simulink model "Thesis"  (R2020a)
settings: Solver=ode15s  StartTime=0.0  StopTime=1440  MaxStep=1  RelTol=1e-3
model workspace (MAT data in the model file):
  SDO_OutputTimes = [0 45 72 95 129 186 320 430 960 1290]
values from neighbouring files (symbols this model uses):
  BR = 5000    [VariablesHighBFloretsSR.m]    (also in VariablesHighBPowderSR.m; VariablesLowBFloretsSR.m; VariablesMedBFloretsSR.m; VariablesNoBFloretsSR.m)
  Cgl0 = 621.875    [VariablesHighBFloretsSR.m]    (also in VariablesHighBPowderSR.m = 383.33; VariablesLowBFloretsSR.m = 708.333; VariablesMedBFloretsSR.m = 667.70833; VariablesNoBFloretsSR.m = 734.375)
  ITC0 = 115.625    [VariablesHighBFloretsSR.m]    (also in VariablesHighBPowderSR.m = 354.17; VariablesLowBFloretsSR.m = 2.65154545455; VariablesMedBFloretsSR.m = 2.40689655172; VariablesNoBFloretsSR.m = 3.125)
  ka = 0.17952    [VariablesHighBFloretsSR.m]    (also in VariablesHighBPowderSR.m; VariablesLowBFloretsSR.m; VariablesMedBFloretsSR.m; VariablesNoBFloretsSR.m)
  ke = 0.024    [VariablesHighBFloretsSR.m]    (also in VariablesHighBPowderSR.m; VariablesLowBFloretsSR.m; VariablesMedBFloretsSR.m; VariablesNoBFloretsSR.m)
  keni = 0.0015    [VariablesHighBFloretsSR.m]    (also in VariablesHighBPowderSR.m; VariablesLowBFloretsSR.m; VariablesMedBFloretsSR.m; VariablesNoBFloretsSR.m)
  kf = 0.00333    [VariablesHighBFloretsSR.m]    (also in VariablesHighBPowderSR.m; VariablesLowBFloretsSR.m; VariablesMedBFloretsSR.m; VariablesNoBFloretsSR.m)
  Ki = 893.018606646    [VariablesHighBFloretsSR.m]    (also in VariablesHighBPowderSR.m; VariablesLowBFloretsSR.m; VariablesMedBFloretsSR.m; VariablesNoBFloretsSR.m)
  Km = 110.161136443    [VariablesHighBFloretsSR.m]    (also in VariablesHighBPowderSR.m; VariablesLowBFloretsSR.m; VariablesMedBFloretsSR.m; VariablesNoBFloretsSR.m)
  ktli = 0.002682    [VariablesHighBFloretsSR.m]    (also in VariablesHighBPowderSR.m; VariablesLowBFloretsSR.m; VariablesMedBFloretsSR.m; VariablesNoBFloretsSR.m)
  ktsi = 0.03518    [VariablesHighBFloretsSR.m]    (also in VariablesHighBPowderSR.m; VariablesLowBFloretsSR.m; VariablesMedBFloretsSR.m; VariablesNoBFloretsSR.m = 0.0351)
  M = 30    [VariablesHighBFloretsSR.m]    (also in VariablesHighBPowderSR.m; VariablesLowBFloretsSR.m; VariablesMedBFloretsSR.m; VariablesNoBFloretsSR.m)
  MYR = 0.0348960299    [VariablesHighBFloretsSR.m]    (also in VariablesHighBPowderSR.m; VariablesLowBFloretsSR.m = 0.000562839; VariablesMedBFloretsSR.m = 0.006528935; VariablesNoBFloretsSR.m = 1.12568e-05)
  NLI = 7    [VariablesHighBFloretsSR.m]    (also in VariablesHighBPowderSR.m; VariablesLowBFloretsSR.m; VariablesMedBFloretsSR.m; VariablesNoBFloretsSR.m)
  NSI = 6    [VariablesHighBFloretsSR.m]    (also in VariablesHighBPowderSR.m; VariablesLowBFloretsSR.m; VariablesMedBFloretsSR.m; VariablesNoBFloretsSR.m)
  SH = 0.02    [VariablesHighBFloretsSR.m]    (also in VariablesHighBPowderSR.m; VariablesLowBFloretsSR.m; VariablesMedBFloretsSR.m; VariablesNoBFloretsSR.m)
  SRR = 0.4737    [VariablesHighBFloretsSR.m]    (also in VariablesHighBPowderSR.m; VariablesLowBFloretsSR.m; VariablesMedBFloretsSR.m; VariablesNoBFloretsSR.m)
  St = 30    [VariablesHighBFloretsSR.m]    (also in VariablesHighBPowderSR.m; VariablesLowBFloretsSR.m; VariablesMedBFloretsSR.m; VariablesNoBFloretsSR.m)
  V1 = 0.096    [VariablesHighBFloretsSR.m]    (also in VariablesHighBPowderSR.m; VariablesLowBFloretsSR.m; VariablesMedBFloretsSR.m; VariablesNoBFloretsSR.m)
  V18 = 5    [VariablesHighBFloretsSR.m]    (also in VariablesHighBPowderSR.m; VariablesLowBFloretsSR.m; VariablesMedBFloretsSR.m; VariablesNoBFloretsSR.m)
  V2 = 0.05    [VariablesHighBFloretsSR.m]    (also in VariablesHighBPowderSR.m; VariablesLowBFloretsSR.m; VariablesMedBFloretsSR.m; VariablesNoBFloretsSR.m)
  V3 = 0.15    [VariablesHighBFloretsSR.m]    (also in VariablesHighBPowderSR.m; VariablesLowBFloretsSR.m; VariablesMedBFloretsSR.m; VariablesNoBFloretsSR.m)
  V4 = 0.2    [VariablesHighBFloretsSR.m]    (also in VariablesHighBPowderSR.m; VariablesLowBFloretsSR.m; VariablesMedBFloretsSR.m; VariablesNoBFloretsSR.m)
  VLI = 3.4    [VariablesHighBFloretsSR.m]    (also in VariablesHighBPowderSR.m; VariablesLowBFloretsSR.m; VariablesMedBFloretsSR.m; VariablesNoBFloretsSR.m)
  Vmax = 2070    [VariablesHighBFloretsSR.m]    (also in VariablesHighBPowderSR.m; VariablesLowBFloretsSR.m; VariablesMedBFloretsSR.m; VariablesNoBFloretsSR.m)
  VSI = 1.5    [VariablesHighBFloretsSR.m]    (also in VariablesHighBPowderSR.m; VariablesLowBFloretsSR.m; VariablesMedBFloretsSR.m; VariablesNoBFloretsSR.m)
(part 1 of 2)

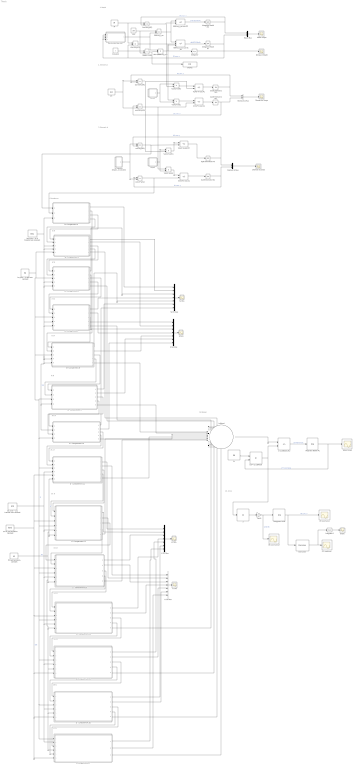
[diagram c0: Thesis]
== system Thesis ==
  note: 1. Mouth
  note: 2. Stomach a
  note: 3. Stomach b
  note: 4. Duodenum
  note: 5. SI
  note: 6. SI
  note: 7. SI
  note: 8. SI
  note: 9. SI
  note: 10. SI
  note: 11. LI
  note: 12. LI
  note: 13. LI
  note: 14. LI
  note: 15. LI
  note: 16. LI
  note: 17. LI
  note: 18. Blood
  note: 19. Urine
  -SRR*myr_rxn-out-nit,GL : Sum  Inputs=|---
  Blood Scope : Scope
  CL : Constant  Value=ke
  Constant : Constant
  Derivative : Derivative
  Display : Display
  Gain1 : Gain  Gain=V18
  ITC conc Urine : Scope
  ITC conc Urine2 : Scope
  ITC gut formation constant : Constant  Value=kf
  "ITC umol/min " : Scope
  In Blood : Sum  Inputs=|+++++++++++++
  Integrator : Integrator
  Integrator Blood ITC : Integrator
  Integrator Mouth GL : Integrator  InitialCondition=Cgl0
  Integrator Mouth ITC : Integrator  InitialCondition=ITC0
  Integrator Urine : Integrator
  Integrator1 : Integrator
  LI - Compartment 11 : Subsystem
  LI - Compartment 12 : Subsystem
  LI - Compartment 13 : Subsystem
  LI - Compartment 14 : Subsystem
  LI - Compartment 15 : Subsystem
  LI - Compartment 16 : Subsystem
  LI Compartment 17 : Subsystem
  LI GL Mux : Mux  Inputs=7
  LI GLs : Scope
  LI ITC Mux : Mux  Inputs=7
  LI ITCs : Scope
  M : Constant  Value=M
  Mouth Mux : Mux  Inputs=2
  Mouth Scope : Scope
  "Myrosinase Reaction " : Subsystem
  Nit=SRNR*myr_rxn : Product
  Nitriles in Mouth : Scope
  Out=M*y(GL) : Product
  Out=M*y(ITC) : Product
  "S, stomach emptying rate constant" : Subsystem
  SH : Constant  Value=SH
  SI - Compartment 10 : Subsystem
  SI - Compartment 5 : Subsystem
  SI - Compartment 6 : Subsystem
  SI - Compartment 7 : Subsystem
  SI - Compartment 8 : Subsystem
  SI - Compartment 9 : Subsystem
  SI GL Mux : Mux  Inputs=7
  SI GLs : Scope
  SI ITC Mux : Mux  Inputs=7
  SI ITCs : Scope
  "SI- Compartment 4 " : Subsystem
  SRNR=1-SRR : Sum  Inputs=+-
  SRR : Constant  Value=SRR
  SRR*myr_rxn : Product
  SRR*myr_rxn-out,ITC : Sum  Inputs=|+-
  Scope : Scope
  Stomach a Mux : Mux  Inputs=2
  Stomach a Scope : Scope
  Stomach b Mux : Mux  Inputs=2
  Stomach b Scope : Scope
  V1/V2 : Subsystem
  V1/V2*in(GL) : Product
  V1/V2*in(ITC) : Product
  V1/V2*in-out,GL : Sum  Inputs=|+-
  V1/V2*in-out,ITC : Sum  Inputs=+-
  V2/V3 : Subsystem
  V2/V3*in(GL) : Product
  V2/V3*in(ITC) : Product
  V2/V3*in-out,GL : Sum  Inputs=|+-
  V2/V3*in-out,ITC : Sum  Inputs=+-
  dy/dt Stomach1 GL1 : Integrator
  dy/dt Stomach1 ITC1 : Integrator
  dy/dt Stomach2 GL : Integrator
  dy/dt Stomach2 ITC : Integrator
  eru-ni gut formation constant : Constant  Value=keni
  in : Product  Inputs=1
  in-out(Blood,ITC) : Sum  Inputs=|+-
  ka,(min^-1) abs rate constant : Constant  Value=ka
  ktli,(min^-1) LI transfer rate constant : Constant  Value=ktli
  ktsi,(min^-1) SI transfer rate constant : Constant  Value=ktsi
  out= CL*y(Blood) : Product
  out=S*y(GL) : Product
  out=S*y(ITC) : Product
  out=SH*y(GL) : Product
  out=SH*y(ITC) : Product
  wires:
  Integrator Mouth ITC/1 -> Mouth Mux/1, Out=M*y(ITC)/2  "ITC conc, y"
  Integrator Mouth GL/1 -> Mouth Mux/2, Out=M*y(GL)/2, "Myrosinase Reaction "/1("GL conc, y"), "Myrosinase Reaction "/2("GL conc, y1"), "Myrosinase Reaction "/3("GL conc, y2")  "GL conc, y"
  Mouth Mux/1 -> Mouth Scope/1
  M/1 -> Out=M*y(GL)/1, Out=M*y(ITC)/1
  Out=M*y(ITC)/1 -> V1/V2*in(ITC)/2, SRR*myr_rxn-out,ITC/2
  "Myrosinase Reaction "/1(Out1) -> Nit=SRNR*myr_rxn/1, SRR*myr_rxn/2
  Out=M*y(GL)/1 -> -SRR*myr_rxn-out-nit,GL/2, V1/V2*in(GL)/1
  SRR*myr_rxn-out,ITC/1 -> Integrator Mouth ITC/1  "dy/dt ITC Mouth"
  -SRR*myr_rxn-out-nit,GL/1 -> Integrator Mouth GL/1  "dy/dt GL Mouth"
  SH/1 -> out=SH*y(ITC)/1, out=SH*y(GL)/2
  Stomach a Mux/1 -> Stomach a Scope/1
  dy/dt Stomach1 GL1/1 -> out=SH*y(GL)/1, Stomach a Mux/2  "GL conc, y"
  dy/dt Stomach1 ITC1/1 -> Stomach a Mux/1, out=SH*y(ITC)/2  "ITC conc, y"
  V1/V2/1(Out1) -> V1/V2*in(ITC)/1, V1/V2*in(GL)/2
  V1/V2*in(GL)/1 -> V1/V2*in-out,GL/1
  V1/V2*in(ITC)/1 -> V1/V2*in-out,ITC/1
  V1/V2*in-out,ITC/1 -> dy/dt Stomach1 ITC1/1
  V1/V2*in-out,GL/1 -> dy/dt Stomach1 GL1/1
  dy/dt Stomach2 GL/1 -> Stomach b Mux/2, out=S*y(GL)/1  "GL conc, y"
  V2/V3*in(ITC)/1 -> V2/V3*in-out,ITC/1
  out=SH*y(ITC)/1 -> V1/V2*in-out,ITC/2, V2/V3*in(ITC)/2
  dy/dt Stomach2 ITC/1 -> out=S*y(ITC)/2, Stomach b Mux/1  "ITC conc, y"
  out=SH*y(GL)/1 -> V2/V3*in(GL)/1, V1/V2*in-out,GL/2
  V2/V3*in(GL)/1 -> V2/V3*in-out,GL/1
  Stomach b Mux/1 -> Stomach b Scope/1
  V2/V3*in-out,GL/1 -> dy/dt Stomach2 GL/1
  V2/V3/1(Out1) -> V2/V3*in(ITC)/1, V2/V3*in(GL)/2
  V2/V3*in-out,ITC/1 -> dy/dt Stomach2 ITC/1
  "S, stomach emptying rate constant"/1(Out1) -> out=S*y(ITC)/1, out=S*y(GL)/2
  out=S*y(GL)/1 -> "SI- Compartment 4 "/2(In GL), V2/V3*in-out,GL/2
  out=S*y(ITC)/1 -> "SI- Compartment 4 "/1(In ITC), V2/V3*in-out,ITC/2
  SI ITC Mux/1 -> SI ITCs/1
  SI GL Mux/1 -> SI GLs/1
  "SI- Compartment 4 "/1("ITC conc, y") -> SI ITC Mux/1
  "SI- Compartment 4 "/2("GL conc, y") -> SI GL Mux/1
  "SI- Compartment 4 "/3(Out ITC) -> SI - Compartment 5/1(In ITC)
  "SI- Compartment 4 "/4(Out GL) -> SI - Compartment 5/2(In GL)
  SI - Compartment 5/1("ITC conc, y") -> SI ITC Mux/2
  SI - Compartment 5/2("GL conc, y") -> SI GL Mux/2
  SI - Compartment 5/3(Out ITC) -> SI - Compartment 6/1(In ITC)
  SI - Compartment 5/4(Out GL) -> SI - Compartment 6/2(In GL)
  SI - Compartment 6/1("ITC conc, y") -> SI ITC Mux/3
  SI - Compartment 6/2("GL conc, y") -> SI GL Mux/3
  SI - Compartment 6/3(Out ITC) -> SI - Compartment 7/1(In ITC)
  SI - Compartment 6/4(Out GL) -> SI - Compartment 7/2(In GL)
  SI - Compartment 7/1("ITC conc, y") -> SI ITC Mux/4
  SI - Compartment 7/2("GL conc, y") -> SI GL Mux/4
  ktsi,(min^-1) SI transfer rate constant/1 -> "SI- Compartment 4 "/3(ktsi), SI - Compartment 8/4(ktsi), SI - Compartment 10/2(ktsi), SI - Compartment 9/4(ktsi), SI - Compartment 8/5(ktsi1), SI - Compartment 7/5(ktsi GL), SI - Compartment 7/4(ktsi ITC), SI - Compartment 6/5(ktsi GL), SI - Compartment 6/4(ktsi ITC), SI - Compartment 5/4(ktsi GL), SI - Compartment 5/3(ktsi ITC)  "ktsi"
  SI - Compartment 7/3(Out ITC) -> SI - Compartment 8/1(In ITC)
  SI - Compartment 7/4(Out GL) -> SI - Compartment 8/2(In GL)
  SI - Compartment 8/1("ITC conc, y") -> SI ITC Mux/5
  SI - Compartment 8/2("GL conc, y") -> SI GL Mux/5
  SI - Compartment 8/3(Out ITC) -> SI - Compartment 9/1(In ITC)
  SI - Compartment 8/4(Out GL) -> SI - Compartment 9/2(In GL)
  SI - Compartment 9/1("ITC conc, y") -> SI ITC Mux/6
  SI - Compartment 9/2("GL conc, y") -> SI GL Mux/6
  LI GL Mux/1 -> LI GLs/1
  LI ITC Mux/1 -> LI ITCs/1
  SI - Compartment 9/3(Out ITC) -> SI - Compartment 10/1(In ITC)
  SI - Compartment 9/4(Out GL) -> SI - Compartment 10/3(In GL)
  SI - Compartment 10/1("ITC conc, y") -> SI ITC Mux/7
  SI - Compartment 10/2("GL conc, y") -> SI GL Mux/7
  SI - Compartment 10/3(Out ITC) -> LI - Compartment 11/1(In ITC)
  SI - Compartment 10/4(Out GL) -> LI - Compartment 11/2(In GL)
  LI - Compartment 11/1("ITC conc, y") -> LI ITC Mux/1
  LI - Compartment 11/2("GL conc, y") -> LI GL Mux/1
  LI - Compartment 11/3(Out ITC) -> LI - Compartment 12/1(In1)
  LI - Compartment 11/4(Out GL) -> LI - Compartment 12/2(In2)
  LI - Compartment 12/1("ITC conc, y") -> LI ITC Mux/2
  LI - Compartment 12/2("GL conc, y") -> LI GL Mux/2
  ktli,(min^-1) LI transfer rate constant/1 -> LI - Compartment 14/5(ktli), LI Compartment 17/2(ktli), LI - Compartment 16/4(ktli), LI - Compartment 15/4(ktli), LI - Compartment 13/5(ktli), LI - Compartment 12/5(ktli), LI - Compartment 11/4(ktli)  "ktli"
  ka,(min^-1) abs rate constant/1 -> SI - Compartment 7/3(ka), LI Compartment 17/1(ka), LI - Compartment 16/3(ka), LI - Compartment 15/3(ka), LI - Compartment 14/4(ka), LI - Compartment 13/4(ka), LI - Compartment 12/4(ka), LI - Compartment 11/3(ka), SI - Compartment 10/4(ka), SI - Compartment 9/3(ka), SI - Compartment 8/3(ka), SI - Compartment 6/3(ka), SI - Compartment 5/5(Ka)  "ka"
  eru-ni gut formation constant/1 -> LI Compartment 17/6(keni), LI - Compartment 16/6(keni), LI - Compartment 15/6(keni), LI - Compartment 14/3(keni), LI - Compartment 13/3(keni), LI - Compartment 11/5(keni), LI - Compartment 12/3(keni)  "keni"
  ITC gut formation constant/1 -> LI - Compartment 12/6(kf), LI - Compartment 11/6(kf), LI Compartment 17/4(kf), LI - Compartment 16/5(kf), LI - Compartment 15/5(kf), LI - Compartment 14/6(kf), LI - Compartment 13/6(kf)  "kf"
  LI - Compartment 12/3(Out ITC) -> LI - Compartment 13/1(In1)
  LI - Compartment 12/4(Out GL) -> LI - Compartment 13/2(In2)
  LI - Compartment 13/1("ITC conc, y") -> LI ITC Mux/3
  LI - Compartment 13/2("GL conc, y") -> LI GL Mux/3
  LI - Compartment 13/3(Out ITC) -> LI - Compartment 14/1(In1)
  LI - Compartment 13/4(Out GL) -> LI - Compartment 14/2(In2)
  LI - Compartment 14/1("ITC conc, y") -> LI ITC Mux/4
  LI - Compartment 14/2("GL conc, y") -> LI GL Mux/4
  LI - Compartment 14/3(Out ITC) -> LI - Compartment 15/1(In1)
  LI - Compartment 14/4(Out GL) -> LI - Compartment 15/2(In2)
  LI - Compartment 15/1("ITC conc, y") -> LI ITC Mux/5
  LI - Compartment 15/2("GL conc, y") -> LI GL Mux/5
  LI - Compartment 15/3(Out ITC) -> LI - Compartment 16/1(In1)
  LI - Compartment 15/4(Out GL) -> LI - Compartment 16/2(In2)
  LI - Compartment 16/1("ITC conc, y") -> LI ITC Mux/6
  LI - Compartment 16/2("GL conc, y") -> LI GL Mux/6
  LI - Compartment 16/3(Out ITC) -> LI Compartment 17/3(In3)
  LI - Compartment 16/4(Out GL) -> LI Compartment 17/5(In5)
  LI Compartment 17/1("ITC conc, y") -> LI ITC Mux/7
  LI Compartment 17/2("GL conc, y") -> LI GL Mux/7
  SI - Compartment 5/5(abs) -> In Blood/1
  SI - Compartment 6/5(abs) -> In Blood/2
  SI - Compartment 7/5(abs) -> In Blood/3
  SI - Compartment 8/5(abs) -> In Blood/4
  SI - Compartment 9/5(abs) -> In Blood/5
  SI - Compartment 10/5(abs) -> In Blood/6
  LI - Compartment 11/5(abs) -> In Blood/7
  LI - Compartment 12/5(abs) -> In Blood/8
  LI - Compartment 13/5(abs) -> In Blood/9
  LI - Compartment 14/5(abs) -> In Blood/10
  LI - Compartment 15/5(abs) -> In Blood/11
  LI Compartment 17/3(abs) -> In Blood/13
  In Blood/1 -> in-out(Blood,ITC)/1
  CL/1 -> out= CL*y(Blood)/1
  Integrator Blood ITC/1 -> Blood Scope/1, out= CL*y(Blood)/2  "ITC conc Blood"
  out= CL*y(Blood)/1 -> in-out(Blood,ITC)/2, in/1
  in-out(Blood,ITC)/1 -> Integrator Blood ITC/1  "dy/dt Blood ITC"
  in/1 -> Gain1/1
  Integrator Urine/1 -> Derivative/1, ITC conc Urine/1  "ITC conc, y"
  LI - Compartment 16/5(abs) -> In Blood/12
  Gain1/1 -> ITC conc Urine2/1, Integrator Urine/1  "umol ITC"
  Derivative/1 -> Integrator1/1, "ITC umol/min "/1
  Nit=SRNR*myr_rxn/1 -> -SRR*myr_rxn-out-nit,GL/3, Integrator/1
  Integrator/1 -> Nitriles in Mouth/1
  Integrator1/1 -> Scope/1
  SRR/1 -> SRR*myr_rxn/1, SRNR=1-SRR/2
  SRR*myr_rxn/1 -> SRR*myr_rxn-out,ITC/1, -SRR*myr_rxn-out-nit,GL/1
  Constant/1 -> SRNR=1-SRR/1
  SRNR=1-SRR/1 -> Display/1, Nit=SRNR*myr_rxn/2

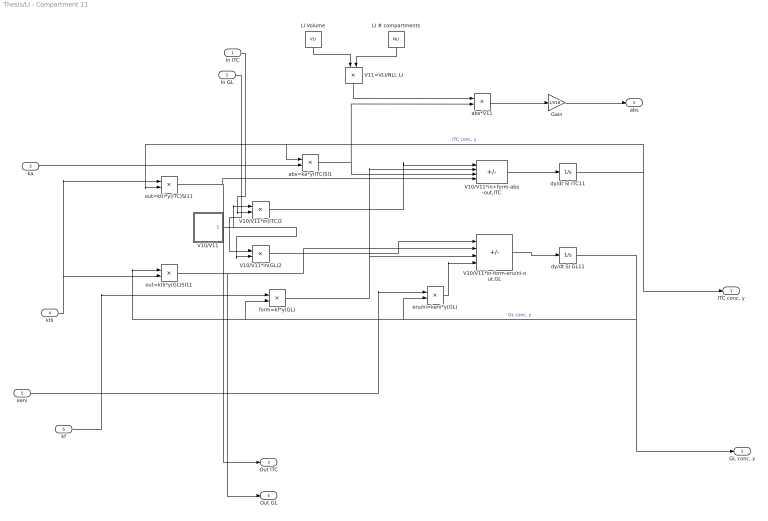
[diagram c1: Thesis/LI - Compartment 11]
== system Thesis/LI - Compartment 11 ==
  In ITC : Inport
  In GL : Inport  Port=2
  ka : Inport  Port=3
  ktli : Inport  Port=4
  keni : Inport  Port=5
  kf : Inport  Port=6
  Gain : Gain  Gain=1/V18
  LI # compartments : Constant  Value=NLI
  LI Volume : Constant  Value=VLI
  V10/V11 : Subsystem
  V10/V11*in(GL)2 : Product
  V10/V11*in(ITC)2 : Product
  V10/V11*in+form-abs-out,ITC : Sum  Inputs=++--
  V10/V11*in-form-eru/ni-out,GL : Sum  Inputs=|+---
  "V11=VLI/NLI, LI " : Product  Inputs=*/
  abs*V11 : Product
  abs=ka*y(ITC)SI1 : Product
  dy/dt SI GL11 : Integrator
  dy/dt SI ITC11 : Integrator
  eru/ni=keni*y(GL) : Product
  form=kf*y(GL) : Product
  out=ktli*y(GL)SI11 : Product
  out=ktli*y(ITC)SI11 : Product
  "ITC conc, y" : Outport
  "GL conc, y" : Outport  Port=2
  Out ITC : Outport  Port=3
  Out GL : Outport  Port=4
  abs : Outport  Port=5
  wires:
  dy/dt SI ITC11/1 -> "ITC conc, y"/1, abs=ka*y(ITC)SI1/1, out=ktli*y(ITC)SI11/2  "ITC conc, y"
  abs=ka*y(ITC)SI1/1 -> abs*V11/2, V10/V11*in+form-abs-out,ITC/3
  out=ktli*y(GL)SI11/1 -> Out GL/1, V10/V11*in-form-eru/ni-out,GL/2
  V10/V11*in-form-eru/ni-out,GL/1 -> dy/dt SI GL11/1
  dy/dt SI GL11/1 -> form=kf*y(GL)/2, out=ktli*y(GL)SI11/1, eru/ni=keni*y(GL)/2, "GL conc, y"/1  "GL conc, y"
  ktli/1 -> out=ktli*y(GL)SI11/2, out=ktli*y(ITC)SI11/1
  V10/V11*in(GL)2/1 -> V10/V11*in-form-eru/ni-out,GL/1
  V10/V11/1(Out1) -> V10/V11*in(GL)2/2, V10/V11*in(ITC)2/1
  form=kf*y(GL)/1 -> V10/V11*in+form-abs-out,ITC/2, V10/V11*in-form-eru/ni-out,GL/3
  V10/V11*in(ITC)2/1 -> V10/V11*in+form-abs-out,ITC/1
  V10/V11*in+form-abs-out,ITC/1 -> dy/dt SI ITC11/1
  eru/ni=keni*y(GL)/1 -> V10/V11*in-form-eru/ni-out,GL/4
  out=ktli*y(ITC)SI11/1 -> Out ITC/1, V10/V11*in+form-abs-out,ITC/4
  ka/1 -> abs=ka*y(ITC)SI1/2
  In ITC/1 -> V10/V11*in(ITC)2/2
  In GL/1 -> V10/V11*in(GL)2/1
  keni/1 -> eru/ni=keni*y(GL)/1
  kf/1 -> form=kf*y(GL)/1
  LI Volume/1 -> "V11=VLI/NLI, LI "/1
  LI # compartments/1 -> "V11=VLI/NLI, LI "/2
  "V11=VLI/NLI, LI "/1 -> abs*V11/1
  abs*V11/1 -> Gain/1
  Gain/1 -> abs/1

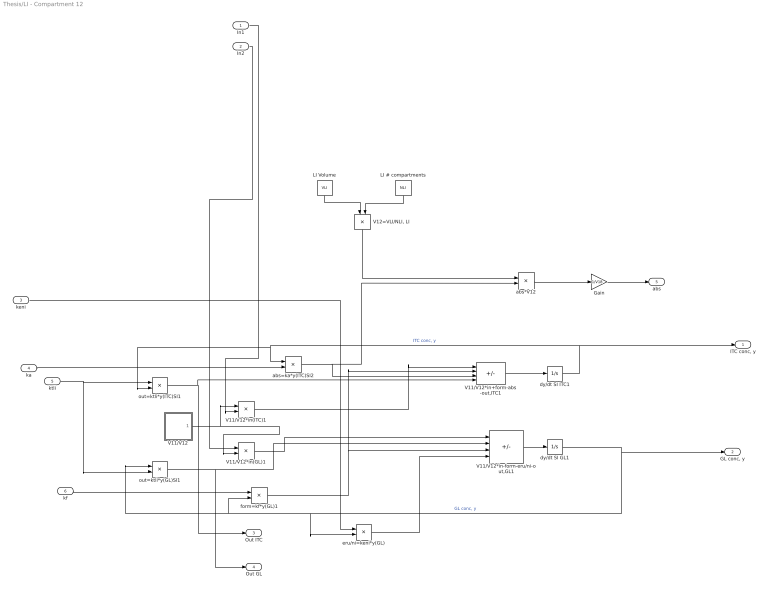
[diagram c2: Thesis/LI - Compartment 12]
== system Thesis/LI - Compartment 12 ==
  In1 : Inport
  In2 : Inport  Port=2
  keni : Inport  Port=3
  ka : Inport  Port=4
  ktli : Inport  Port=5
  kf : Inport  Port=6
  Gain : Gain  Gain=1/V18
  LI # compartments : Constant  Value=NLI
  LI Volume : Constant  Value=VLI
  V11/V12 : Subsystem
  V11/V12*in(GL)1 : Product
  V11/V12*in(ITC)1 : Product
  V11/V12*in+form-abs-out,ITC1 : Sum  Inputs=++--
  V11/V12*in-form-eru/ni-out,GL1 : Sum  Inputs=|+---
  "V12=VLI/NLI, LI " : Product  Inputs=*/
  abs*V12 : Product
  abs=ka*y(ITC)SI2 : Product
  dy/dt SI GL1 : Integrator
  dy/dt SI ITC1 : Integrator
  eru/ni=keni*y(GL) : Product
  form=kf*y(GL)1 : Product
  out=ktli*y(GL)SI1 : Product
  out=ktli*y(ITC)SI1 : Product
  "ITC conc, y" : Outport
  "GL conc, y" : Outport  Port=2
  Out ITC : Outport  Port=3
  Out GL : Outport  Port=4
  abs : Outport  Port=5
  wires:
  In2/1 -> V11/V12*in(GL)1/1
  dy/dt SI GL1/1 -> "GL conc, y"/1, form=kf*y(GL)1/2, out=ktli*y(GL)SI1/1, eru/ni=keni*y(GL)/2  "GL conc, y"
  V11/V12/1(Out1) -> V11/V12*in(GL)1/2, V11/V12*in(ITC)1/1
  dy/dt SI ITC1/1 -> "ITC conc, y"/1, abs=ka*y(ITC)SI2/1, out=ktli*y(ITC)SI1/2  "ITC conc, y"
  eru/ni=keni*y(GL)/1 -> V11/V12*in-form-eru/ni-out,GL1/4
  V11/V12*in-form-eru/ni-out,GL1/1 -> dy/dt SI GL1/1
  keni/1 -> eru/ni=keni*y(GL)/1
  V11/V12*in(GL)1/1 -> V11/V12*in-form-eru/ni-out,GL1/1
  ktli/1 -> out=ktli*y(GL)SI1/2, out=ktli*y(ITC)SI1/1
  out=ktli*y(GL)SI1/1 -> Out GL/1, V11/V12*in-form-eru/ni-out,GL1/2
  form=kf*y(GL)1/1 -> V11/V12*in+form-abs-out,ITC1/2, V11/V12*in-form-eru/ni-out,GL1/3
  out=ktli*y(ITC)SI1/1 -> Out ITC/1, V11/V12*in+form-abs-out,ITC1/4
  V11/V12*in+form-abs-out,ITC1/1 -> dy/dt SI ITC1/1
  V11/V12*in(ITC)1/1 -> V11/V12*in+form-abs-out,ITC1/1
  ka/1 -> abs=ka*y(ITC)SI2/2
  In1/1 -> V11/V12*in(ITC)1/2
  kf/1 -> form=kf*y(GL)1/1
  LI # compartments/1 -> "V12=VLI/NLI, LI "/2
  LI Volume/1 -> "V12=VLI/NLI, LI "/1
  abs*V12/1 -> Gain/1
  Gain/1 -> abs/1
  abs=ka*y(ITC)SI2/1 -> abs*V12/2, V11/V12*in+form-abs-out,ITC1/3
  "V12=VLI/NLI, LI "/1 -> abs*V12/1

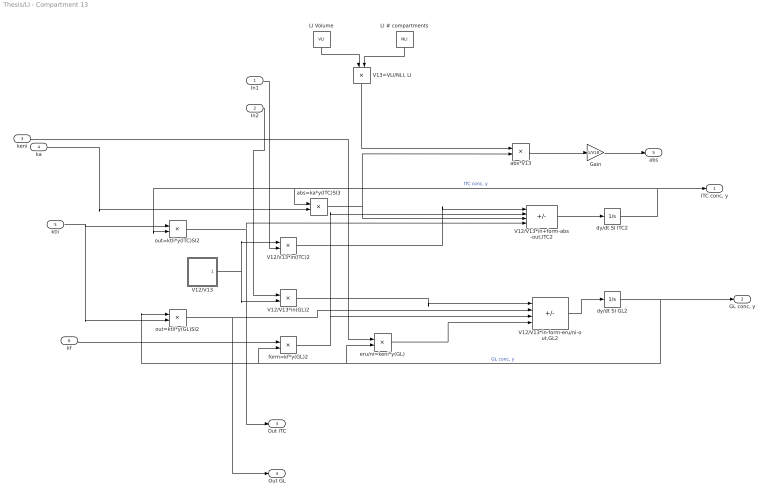
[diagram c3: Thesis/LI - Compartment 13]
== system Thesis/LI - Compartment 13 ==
  In1 : Inport
  In2 : Inport  Port=2
  keni : Inport  Port=3
  ka : Inport  Port=4
  ktli : Inport  Port=5
  kf : Inport  Port=6
  Gain : Gain  Gain=1/V18
  LI # compartments : Constant  Value=NLI
  LI Volume : Constant  Value=VLI
  V12/V13 : Subsystem
  V12/V13*in(GL)2 : Product
  V12/V13*in(ITC)2 : Product
  V12/V13*in+form-abs-out,ITC2 : Sum  Inputs=++--
  V12/V13*in-form-eru/ni-out,GL2 : Sum  Inputs=|+---
  "V13=VLI/NLI, LI " : Product  Inputs=*/
  abs*V13 : Product
  abs=ka*y(ITC)SI3 : Product
  dy/dt SI GL2 : Integrator
  dy/dt SI ITC2 : Integrator
  eru/ni=keni*y(GL) : Product
  form=kf*y(GL)2 : Product
  out=ktli*y(GL)SI2 : Product
  out=ktli*y(ITC)SI2 : Product
  "ITC conc, y" : Outport
  "GL conc, y" : Outport  Port=2
  Out ITC : Outport  Port=3
  Out GL : Outport  Port=4
  abs : Outport  Port=5
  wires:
  dy/dt SI GL2/1 -> "GL conc, y"/1, form=kf*y(GL)2/2, out=ktli*y(GL)SI2/1, eru/ni=keni*y(GL)/2  "GL conc, y"
  eru/ni=keni*y(GL)/1 -> V12/V13*in-form-eru/ni-out,GL2/4
  out=ktli*y(GL)SI2/1 -> Out GL/1, V12/V13*in-form-eru/ni-out,GL2/2
  V12/V13*in(GL)2/1 -> V12/V13*in-form-eru/ni-out,GL2/1
  out=ktli*y(ITC)SI2/1 -> Out ITC/1, V12/V13*in+form-abs-out,ITC2/4
  V12/V13/1(Out1) -> V12/V13*in(GL)2/2, V12/V13*in(ITC)2/1
  keni/1 -> eru/ni=keni*y(GL)/1
  V12/V13*in-form-eru/ni-out,GL2/1 -> dy/dt SI GL2/1
  dy/dt SI ITC2/1 -> abs=ka*y(ITC)SI3/1, out=ktli*y(ITC)SI2/2, "ITC conc, y"/1  "ITC conc, y"
  ka/1 -> abs=ka*y(ITC)SI3/2
  V12/V13*in+form-abs-out,ITC2/1 -> dy/dt SI ITC2/1
  V12/V13*in(ITC)2/1 -> V12/V13*in+form-abs-out,ITC2/1
  form=kf*y(GL)2/1 -> V12/V13*in+form-abs-out,ITC2/2, V12/V13*in-form-eru/ni-out,GL2/3
  In2/1 -> V12/V13*in(GL)2/1
  ktli/1 -> out=ktli*y(GL)SI2/2, out=ktli*y(ITC)SI2/1
  In1/1 -> V12/V13*in(ITC)2/2
  kf/1 -> form=kf*y(GL)2/1
  LI # compartments/1 -> "V13=VLI/NLI, LI "/2
  LI Volume/1 -> "V13=VLI/NLI, LI "/1
  abs*V13/1 -> Gain/1
  Gain/1 -> abs/1
  abs=ka*y(ITC)SI3/1 -> abs*V13/2, V12/V13*in+form-abs-out,ITC2/3
  "V13=VLI/NLI, LI "/1 -> abs*V13/1

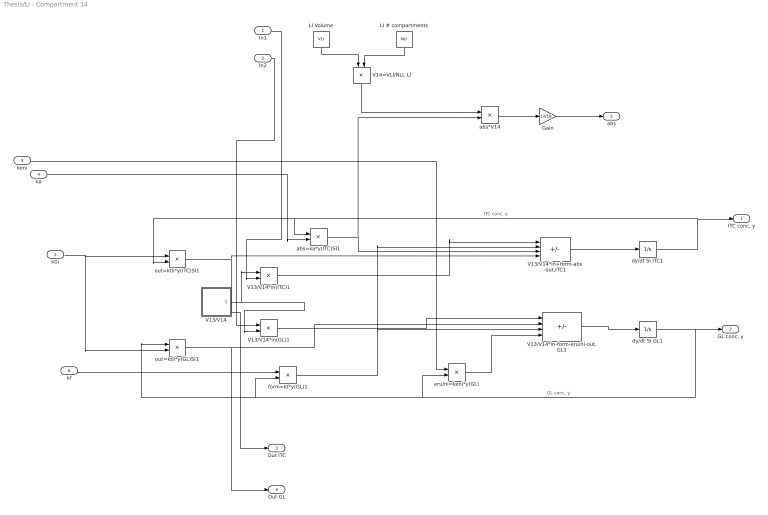
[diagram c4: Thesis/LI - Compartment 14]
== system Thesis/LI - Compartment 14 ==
  In1 : Inport
  In2 : Inport  Port=2
  keni : Inport  Port=3
  ka : Inport  Port=4
  ktli : Inport  Port=5
  kf : Inport  Port=6
  Gain : Gain  Gain=1/V18
  LI # compartments : Constant  Value=NLI
  LI Volume : Constant  Value=VLI
  V13/V14 : Subsystem
  V13/V14*in(GL)1 : Product
  V13/V14*in(ITC)1 : Product
  V13/V14*in+form-abs-out,ITC1 : Sum  Inputs=++--
  V13/V14*in-form-eru/ni-out,GL1 : Sum  Inputs=|+---
  "V14=VLI/NLI, LI " : Product  Inputs=*/
  abs*V14 : Product
  abs=ka*y(ITC)SI1 : Product
  dy/dt SI GL1 : Integrator
  dy/dt SI ITC1 : Integrator
  eru/ni=keni*y(GL) : Product
  form=kf*y(GL)1 : Product
  out=ktli*y(GL)SI1 : Product
  out=ktli*y(ITC)SI1 : Product
  "ITC conc, y" : Outport
  "GL conc, y" : Outport  Port=2
  Out ITC : Outport  Port=3
  Out GL : Outport  Port=4
  abs : Outport  Port=5
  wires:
  V13/V14/1(Out1) -> V13/V14*in(GL)1/2, V13/V14*in(ITC)1/1
  out=ktli*y(GL)SI1/1 -> Out GL/1, V13/V14*in-form-eru/ni-out,GL1/2
  dy/dt SI ITC1/1 -> abs=ka*y(ITC)SI1/1, out=ktli*y(ITC)SI1/2, "ITC conc, y"/1  "ITC conc, y"
  V13/V14*in(ITC)1/1 -> V13/V14*in+form-abs-out,ITC1/1
  out=ktli*y(ITC)SI1/1 -> V13/V14*in+form-abs-out,ITC1/4, Out ITC/1
  form=kf*y(GL)1/1 -> V13/V14*in+form-abs-out,ITC1/2, V13/V14*in-form-eru/ni-out,GL1/3
  eru/ni=keni*y(GL)/1 -> V13/V14*in-form-eru/ni-out,GL1/4
  V13/V14*in+form-abs-out,ITC1/1 -> dy/dt SI ITC1/1
  V13/V14*in(GL)1/1 -> V13/V14*in-form-eru/ni-out,GL1/1
  V13/V14*in-form-eru/ni-out,GL1/1 -> dy/dt SI GL1/1
  dy/dt SI GL1/1 -> "GL conc, y"/1, form=kf*y(GL)1/2, out=ktli*y(GL)SI1/1, eru/ni=keni*y(GL)/2  "GL conc, y"
  In2/1 -> V13/V14*in(GL)1/1
  ka/1 -> abs=ka*y(ITC)SI1/2
  keni/1 -> eru/ni=keni*y(GL)/1
  In1/1 -> V13/V14*in(ITC)1/2
  kf/1 -> form=kf*y(GL)1/1
  ktli/1 -> out=ktli*y(GL)SI1/2, out=ktli*y(ITC)SI1/1
  LI # compartments/1 -> "V14=VLI/NLI, LI "/2
  LI Volume/1 -> "V14=VLI/NLI, LI "/1
  abs*V14/1 -> Gain/1
  Gain/1 -> abs/1
  abs=ka*y(ITC)SI1/1 -> abs*V14/2, V13/V14*in+form-abs-out,ITC1/3
  "V14=VLI/NLI, LI "/1 -> abs*V14/1

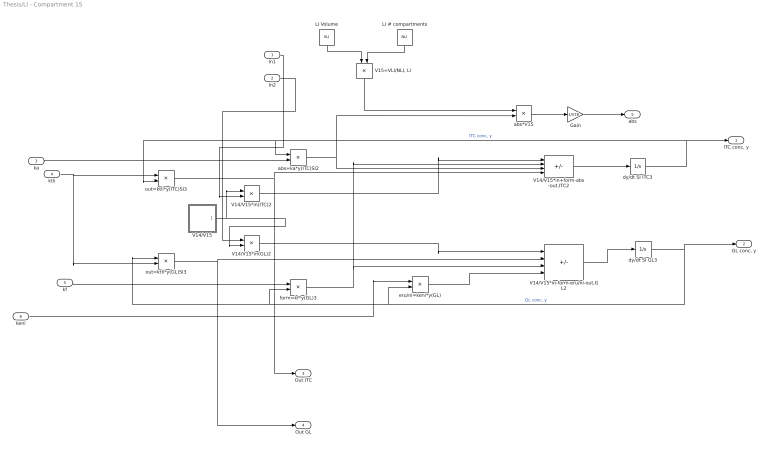
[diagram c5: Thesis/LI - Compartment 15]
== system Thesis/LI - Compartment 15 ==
  In1 : Inport
  In2 : Inport  Port=2
  ka : Inport  Port=3
  ktli : Inport  Port=4
  kf : Inport  Port=5
  keni : Inport  Port=6
  Gain : Gain  Gain=1/V18
  LI # compartments : Constant  Value=NLI
  LI Volume : Constant  Value=VLI
  V14/V15 : Subsystem
  V14/V15*in(GL)2 : Product
  V14/V15*in(ITC)2 : Product
  V14/V15*in+form-abs-out,ITC2 : Sum  Inputs=++--
  V14/V15*in-form-eru/ni-out,GL2 : Sum  Inputs=|+---
  "V15=VLI/NLI, LI " : Product  Inputs=*/
  abs*V15 : Product
  abs=ka*y(ITC)SI2 : Product
  dy/dt SI GL3 : Integrator
  dy/dt SI ITC3 : Integrator
  eru/ni=keni*y(GL) : Product
  form=kf*y(GL)3 : Product
  out=ktli*y(GL)SI3 : Product
  out=ktli*y(ITC)SI3 : Product
  "ITC conc, y" : Outport
  "GL conc, y" : Outport  Port=2
  Out ITC : Outport  Port=3
  Out GL : Outport  Port=4
  abs : Outport  Port=5
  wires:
  In2/1 -> V14/V15*in(GL)2/1
  V14/V15*in(GL)2/1 -> V14/V15*in-form-eru/ni-out,GL2/1
  dy/dt SI GL3/1 -> "GL conc, y"/1, form=kf*y(GL)3/2, out=ktli*y(GL)SI3/1, eru/ni=keni*y(GL)/2  "GL conc, y"
  eru/ni=keni*y(GL)/1 -> V14/V15*in-form-eru/ni-out,GL2/4
  out=ktli*y(GL)SI3/1 -> Out GL/1, V14/V15*in-form-eru/ni-out,GL2/2
  out=ktli*y(ITC)SI3/1 -> Out ITC/1, V14/V15*in+form-abs-out,ITC2/4
  dy/dt SI ITC3/1 -> abs=ka*y(ITC)SI2/1, out=ktli*y(ITC)SI3/2, "ITC conc, y"/1  "ITC conc, y"
  V14/V15/1(Out1) -> V14/V15*in(GL)2/2, V14/V15*in(ITC)2/1
  keni/1 -> eru/ni=keni*y(GL)/1
  V14/V15*in-form-eru/ni-out,GL2/1 -> dy/dt SI GL3/1
  ka/1 -> abs=ka*y(ITC)SI2/2
  V14/V15*in+form-abs-out,ITC2/1 -> dy/dt SI ITC3/1
  form=kf*y(GL)3/1 -> V14/V15*in+form-abs-out,ITC2/2, V14/V15*in-form-eru/ni-out,GL2/3
  kf/1 -> form=kf*y(GL)3/1
  V14/V15*in(ITC)2/1 -> V14/V15*in+form-abs-out,ITC2/1
  ktli/1 -> out=ktli*y(GL)SI3/2, out=ktli*y(ITC)SI3/1
  In1/1 -> V14/V15*in(ITC)2/2
  LI # compartments/1 -> "V15=VLI/NLI, LI "/2
  LI Volume/1 -> "V15=VLI/NLI, LI "/1
  abs*V15/1 -> Gain/1
  Gain/1 -> abs/1
  abs=ka*y(ITC)SI2/1 -> V14/V15*in+form-abs-out,ITC2/3, abs*V15/2
  "V15=VLI/NLI, LI "/1 -> abs*V15/1

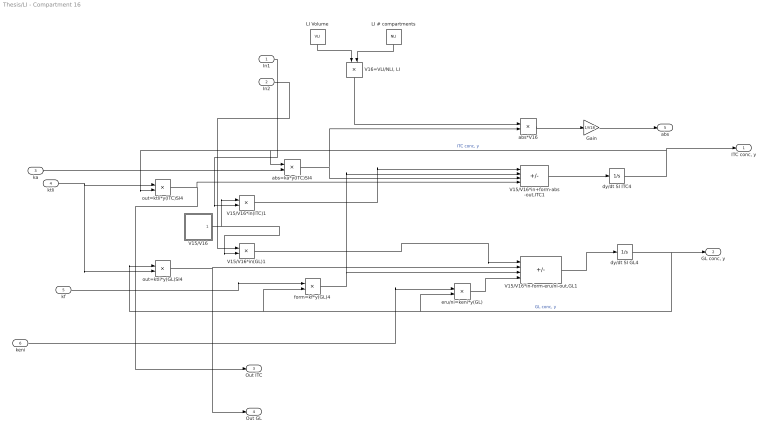
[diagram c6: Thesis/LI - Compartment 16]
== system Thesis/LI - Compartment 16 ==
  In1 : Inport
  In2 : Inport  Port=2
  ka : Inport  Port=3
  ktli : Inport  Port=4
  kf : Inport  Port=5
  keni : Inport  Port=6
  Gain : Gain  Gain=1/V18
  LI # compartments : Constant  Value=NLI
  LI Volume : Constant  Value=VLI
  V15/V16 : Subsystem
  V15/V16*in(GL)1 : Product
  V15/V16*in(ITC)1 : Product
  V15/V16*in+form-abs-out,ITC1 : Sum  Inputs=++--
  V15/V16*in-form-eru/ni-out,GL1 : Sum  Inputs=|+---
  "V16=VLI/NLI, LI " : Product  Inputs=*/
  abs*V16 : Product
  abs=ka*y(ITC)SI4 : Product
  dy/dt SI GL4 : Integrator
  dy/dt SI ITC4 : Integrator
  eru/ni=keni*y(GL) : Product
  form=kf*y(GL)4 : Product
  out=ktli*y(GL)SI4 : Product
  out=ktli*y(ITC)SI4 : Product
  "ITC conc, y" : Outport
  "GL conc, y" : Outport  Port=2
  Out ITC : Outport  Port=3
  Out GL : Outport  Port=4
  abs : Outport  Port=5
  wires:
  out=ktli*y(ITC)SI4/1 -> Out ITC/1, V15/V16*in+form-abs-out,ITC1/4
  out=ktli*y(GL)SI4/1 -> Out GL/1, V15/V16*in-form-eru/ni-out,GL1/2
  dy/dt SI ITC4/1 -> abs=ka*y(ITC)SI4/1, out=ktli*y(ITC)SI4/2, "ITC conc, y"/1  "ITC conc, y"
  V15/V16*in(ITC)1/1 -> V15/V16*in+form-abs-out,ITC1/1
  ka/1 -> abs=ka*y(ITC)SI4/2
  dy/dt SI GL4/1 -> "GL conc, y"/1, form=kf*y(GL)4/2, out=ktli*y(GL)SI4/1, eru/ni=keni*y(GL)/2  "GL conc, y"
  In1/1 -> V15/V16*in(ITC)1/2
  V15/V16/1(Out1) -> V15/V16*in(GL)1/2, V15/V16*in(ITC)1/1
  V15/V16*in+form-abs-out,ITC1/1 -> dy/dt SI ITC4/1
  V15/V16*in-form-eru/ni-out,GL1/1 -> dy/dt SI GL4/1
  keni/1 -> eru/ni=keni*y(GL)/1
  eru/ni=keni*y(GL)/1 -> V15/V16*in-form-eru/ni-out,GL1/4
  V15/V16*in(GL)1/1 -> V15/V16*in-form-eru/ni-out,GL1/1
  form=kf*y(GL)4/1 -> V15/V16*in+form-abs-out,ITC1/2, V15/V16*in-form-eru/ni-out,GL1/3
  In2/1 -> V15/V16*in(GL)1/1
  kf/1 -> form=kf*y(GL)4/1
  ktli/1 -> out=ktli*y(GL)SI4/2, out=ktli*y(ITC)SI4/1
  LI # compartments/1 -> "V16=VLI/NLI, LI "/2
  LI Volume/1 -> "V16=VLI/NLI, LI "/1
  abs*V16/1 -> Gain/1
  Gain/1 -> abs/1
  abs=ka*y(ITC)SI4/1 -> abs*V16/2, V15/V16*in+form-abs-out,ITC1/3
  "V16=VLI/NLI, LI "/1 -> abs*V16/1

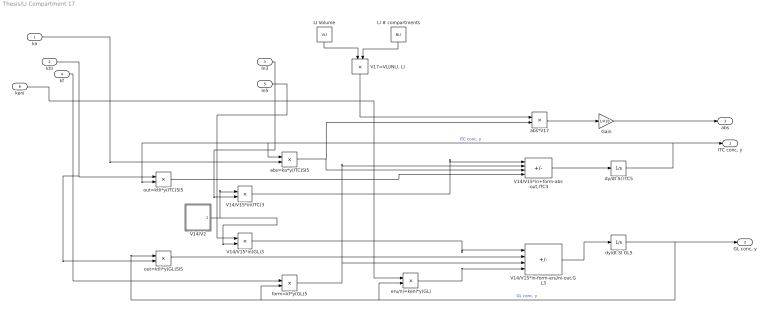
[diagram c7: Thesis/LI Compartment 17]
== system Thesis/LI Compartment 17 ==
  ka : Inport
  ktli : Inport  Port=2
  In3 : Inport  Port=3
  kf : Inport  Port=4
  In5 : Inport  Port=5
  keni : Inport  Port=6
  Gain : Gain  Gain=1/V18
  LI # compartments : Constant  Value=NLI
  LI Volume : Constant  Value=VLI
  V14/V15*in(GL)3 : Product
  V14/V15*in(ITC)3 : Product
  V14/V15*in+form-abs-out,ITC3 : Sum  Inputs=++--
  V14/V15*in-form-eru/ni-out,GL3 : Sum  Inputs=|+---
  V14/V2 : Subsystem
  "V17=VLI/NLI, LI " : Product  Inputs=*/
  abs*V17 : Product
  abs=ka*y(ITC)SI5 : Product
  dy/dt SI GL5 : Integrator
  dy/dt SI ITC5 : Integrator
  eru/ni=keni*y(GL) : Product
  form=kf*y(GL)5 : Product
  out=ktli*y(GL)SI5 : Product
  out=ktli*y(ITC)SI5 : Product
  "ITC conc, y" : Outport
  "GL conc, y" : Outport  Port=2
  abs : Outport  Port=3
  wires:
  dy/dt SI GL5/1 -> "GL conc, y"/1, form=kf*y(GL)5/2, out=ktli*y(GL)SI5/1, eru/ni=keni*y(GL)/2  "GL conc, y"
  form=kf*y(GL)5/1 -> V14/V15*in+form-abs-out,ITC3/2, V14/V15*in-form-eru/ni-out,GL3/3
  V14/V15*in-form-eru/ni-out,GL3/1 -> dy/dt SI GL5/1
  ktli/1 -> out=ktli*y(GL)SI5/2, out=ktli*y(ITC)SI5/1
  V14/V15*in(GL)3/1 -> V14/V15*in-form-eru/ni-out,GL3/1
  eru/ni=keni*y(GL)/1 -> V14/V15*in-form-eru/ni-out,GL3/4
  In3/1 -> V14/V15*in(ITC)3/2
  V14/V2/1(Out1) -> V14/V15*in(GL)3/2, V14/V15*in(ITC)3/1
  out=ktli*y(ITC)SI5/1 -> V14/V15*in+form-abs-out,ITC3/4
  out=ktli*y(GL)SI5/1 -> V14/V15*in-form-eru/ni-out,GL3/2
  V14/V15*in(ITC)3/1 -> V14/V15*in+form-abs-out,ITC3/1
  In5/1 -> V14/V15*in(GL)3/1
  dy/dt SI ITC5/1 -> abs=ka*y(ITC)SI5/1, out=ktli*y(ITC)SI5/2, "ITC conc, y"/1  "ITC conc, y"
  V14/V15*in+form-abs-out,ITC3/1 -> dy/dt SI ITC5/1
  ka/1 -> abs=ka*y(ITC)SI5/2
  keni/1 -> eru/ni=keni*y(GL)/1
  kf/1 -> form=kf*y(GL)5/1
  LI # compartments/1 -> "V17=VLI/NLI, LI "/2
  LI Volume/1 -> "V17=VLI/NLI, LI "/1
  abs*V17/1 -> Gain/1
  Gain/1 -> abs/1
  abs=ka*y(ITC)SI5/1 -> V14/V15*in+form-abs-out,ITC3/3, abs*V17/2
  "V17=VLI/NLI, LI "/1 -> abs*V17/1

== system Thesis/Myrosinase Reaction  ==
  "GL conc, y" : Inport
  "GL conc, y1" : Inport  Port=2
  "GL conc, y2" : Inport  Port=3
  BR : Constant  Value=BR
  Divide : Product  Inputs=*/
  Ki : Constant  Value=Ki
  Km : Constant  Value=Km
  Km+y+y^2/Ki : Sum  Inputs=|+++
  MYR : Constant  Value=MYR
  Vmax : Constant  Value=Vmax
  Vmax*MYR*BR*y : Product  Inputs=4
  y^2 : Math  Operator=square
  y^2/Ki : Product  Inputs=*/
  Out1 : Outport
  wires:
  y^2/1 -> y^2/Ki/1
  MYR/1 -> Vmax*MYR*BR*y/2
  y^2/Ki/1 -> Km+y+y^2/Ki/3
  Divide/1 -> Out1/1
  "GL conc, y2"/1 -> y^2/1
  Km/1 -> Km+y+y^2/Ki/1
  Km+y+y^2/Ki/1 -> Divide/2
  Vmax*MYR*BR*y/1 -> Divide/1
  BR/1 -> Vmax*MYR*BR*y/3
  Vmax/1 -> Vmax*MYR*BR*y/4
  Ki/1 -> y^2/Ki/2
  "GL conc, y"/1 -> Vmax*MYR*BR*y/1
  "GL conc, y1"/1 -> Km+y+y^2/Ki/2

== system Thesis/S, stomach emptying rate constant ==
  Gain : Gain  Gain=-1
  Log : Math  Operator=log  SignedPower=on
  S : Product  Inputs=*/
  St (min),emptying time : Constant  Value=St
  fraction remaining  empty at St : Constant  Value=0.05
  Out1 : Outport
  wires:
  Gain/1 -> S/2
  S/1 -> Out1/1
  fraction remaining  empty at St/1 -> Log/1
  St (min),emptying time/1 -> Gain/1
  Log/1 -> S/1

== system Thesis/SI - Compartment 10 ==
  In ITC : Inport
  ktsi : Inport  Port=2
  In GL : Inport  Port=3
  ka : Inport  Port=4
  Gain : Gain  Gain=1/V18
  SI # compartments : Constant  Value=NSI
  SI Volume : Constant  Value=VSI
  "V10=VSI/NSI, SI " : Product  Inputs=*/
  V9/V10 : Subsystem
  V9/V10*in(GL)1 : Product
  V9/V10*in(ITC)1 : Product
  V9/V10*in-abs-out,ITC : Sum  Inputs=+--
  V9/V10*in-out,GL : Sum  Inputs=|+-
  abs*V10 : Product
  abs=ka*y(ITC)SI10 : Product
  dy/dt SI GL10 : Integrator
  dy/dt SI ITC10 : Integrator
  out=ktsi*y(GL)SI1 : Product
  out=ktsi*y(ITC)SI1 : Product
  "ITC conc, y" : Outport
  "GL conc, y" : Outport  Port=2
  Out ITC : Outport  Port=3
  Out GL : Outport  Port=4
  abs : Outport  Port=5
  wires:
  dy/dt SI GL10/1 -> "GL conc, y"/1, out=ktsi*y(GL)SI1/1  "GL conc, y"
  ktsi/1 -> out=ktsi*y(ITC)SI1/1, out=ktsi*y(GL)SI1/2
  V9/V10*in-abs-out,ITC/1 -> dy/dt SI ITC10/1
  V9/V10*in(ITC)1/1 -> V9/V10*in-abs-out,ITC/1
  out=ktsi*y(GL)SI1/1 -> Out GL/1, V9/V10*in-out,GL/2
  In ITC/1 -> V9/V10*in(ITC)1/2
  V9/V10/1(Out1) -> V9/V10*in(GL)1/2, V9/V10*in(ITC)1/1
  V9/V10*in(GL)1/1 -> V9/V10*in-out,GL/1
  out=ktsi*y(ITC)SI1/1 -> Out ITC/1, V9/V10*in-abs-out,ITC/2
  abs=ka*y(ITC)SI10/1 -> abs*V10/2, V9/V10*in-abs-out,ITC/3
  dy/dt SI ITC10/1 -> out=ktsi*y(ITC)SI1/2, abs=ka*y(ITC)SI10/1, "ITC conc, y"/1  "ITC conc, y"
  V9/V10*in-out,GL/1 -> dy/dt SI GL10/1
  ka/1 -> abs=ka*y(ITC)SI10/2
  In GL/1 -> V9/V10*in(GL)1/1
  SI Volume/1 -> "V10=VSI/NSI, SI "/1
  SI # compartments/1 -> "V10=VSI/NSI, SI "/2
  "V10=VSI/NSI, SI "/1 -> abs*V10/1
  abs*V10/1 -> Gain/1
  Gain/1 -> abs/1

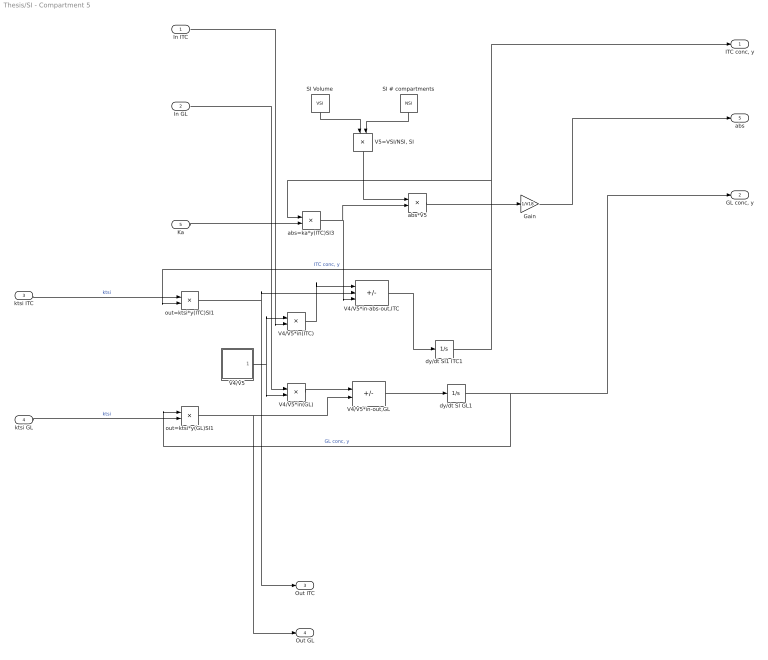
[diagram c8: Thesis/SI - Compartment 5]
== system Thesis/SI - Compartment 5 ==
  In ITC : Inport
  In GL : Inport  Port=2
  ktsi ITC : Inport  Port=3
  ktsi GL : Inport  Port=4
  Ka : Inport  Port=5
  Gain : Gain  Gain=1/V18
  SI # compartments : Constant  Value=NSI
  SI Volume : Constant  Value=VSI
  V4/V5 : Subsystem
  V4/V5*in(GL) : Product
  V4/V5*in(ITC) : Product
  V4/V5*in-abs-out,ITC : Sum  Inputs=+--
  V4/V5*in-out,GL : Sum  Inputs=|+-
  "V5=VSI/NSI, SI " : Product  Inputs=*/
  abs*V5 : Product
  abs=ka*y(ITC)SI3 : Product
  dy/dt SI GL1 : Integrator
  dy/dt SI1 ITC1 : Integrator
  out=ktsi*y(GL)SI1 : Product
  out=ktsi*y(ITC)SI1 : Product
  "ITC conc, y" : Outport
  "GL conc, y" : Outport  Port=2
  Out ITC : Outport  Port=3
  Out GL : Outport  Port=4
  abs : Outport  Port=5
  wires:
  out=ktsi*y(ITC)SI1/1 -> Out ITC/1, V4/V5*in-abs-out,ITC/2
  out=ktsi*y(GL)SI1/1 -> Out GL/1, V4/V5*in-out,GL/2
  V4/V5*in-abs-out,ITC/1 -> dy/dt SI1 ITC1/1
  dy/dt SI GL1/1 -> "GL conc, y"/1, out=ktsi*y(GL)SI1/1  "GL conc, y"
  dy/dt SI1 ITC1/1 -> abs=ka*y(ITC)SI3/1, "ITC conc, y"/1, out=ktsi*y(ITC)SI1/2  "ITC conc, y"
  V4/V5*in-out,GL/1 -> dy/dt SI GL1/1
  V4/V5/1(Out1) -> V4/V5*in(ITC)/1, V4/V5*in(GL)/2
  In GL/1 -> V4/V5*in(GL)/1
  V4/V5*in(GL)/1 -> V4/V5*in-out,GL/1
  V4/V5*in(ITC)/1 -> V4/V5*in-abs-out,ITC/1
  ktsi GL/1 -> out=ktsi*y(GL)SI1/2  "ktsi"
  In ITC/1 -> V4/V5*in(ITC)/2
  ktsi ITC/1 -> out=ktsi*y(ITC)SI1/1  "ktsi"
  Ka/1 -> abs=ka*y(ITC)SI3/2
  abs=ka*y(ITC)SI3/1 -> abs*V5/2, V4/V5*in-abs-out,ITC/3
  abs*V5/1 -> Gain/1
  SI # compartments/1 -> "V5=VSI/NSI, SI "/2
  SI Volume/1 -> "V5=VSI/NSI, SI "/1
  "V5=VSI/NSI, SI "/1 -> abs*V5/1
  Gain/1 -> abs/1

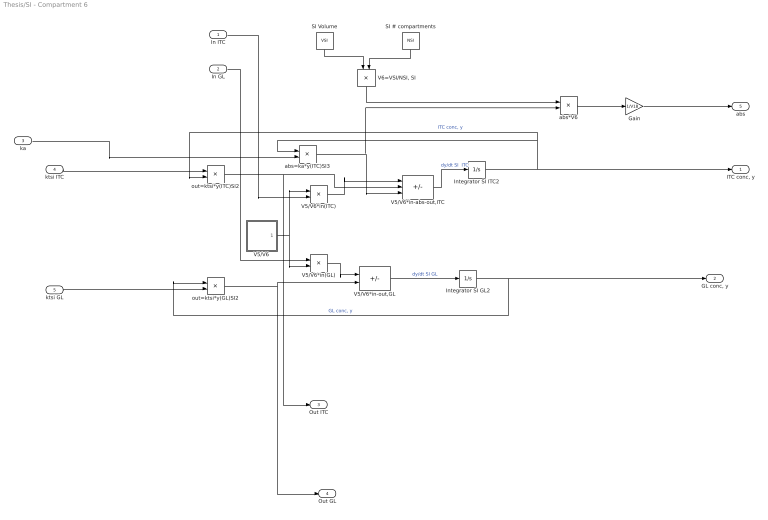
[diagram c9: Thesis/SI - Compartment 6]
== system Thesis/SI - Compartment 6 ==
  In ITC : Inport
  In GL : Inport  Port=2
  ka : Inport  Port=3
  ktsi ITC : Inport  Port=4
  ktsi GL : Inport  Port=5
  Gain : Gain  Gain=1/V18
  Integrator SI GL2 : Integrator
  Integrator SI ITC2 : Integrator
  SI # compartments : Constant  Value=NSI
  SI Volume : Constant  Value=VSI
  V5/V6 : Subsystem
  V5/V6*in(GL) : Product
  V5/V6*in(ITC) : Product
  V5/V6*in-abs-out,ITC : Sum  Inputs=+--
  V5/V6*in-out,GL : Sum  Inputs=|+-
  "V6=VSI/NSI, SI " : Product  Inputs=*/
  abs*V6 : Product
  abs=ka*y(ITC)SI3 : Product
  out=ktsi*y(GL)SI2 : Product
  out=ktsi*y(ITC)SI2 : Product
  "ITC conc, y" : Outport
  "GL conc, y" : Outport  Port=2
  Out ITC : Outport  Port=3
  Out GL : Outport  Port=4
  abs : Outport  Port=5
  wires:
  out=ktsi*y(GL)SI2/1 -> Out GL/1, V5/V6*in-out,GL/2
  abs=ka*y(ITC)SI3/1 -> abs*V6/2, V5/V6*in-abs-out,ITC/3
  V5/V6/1(Out1) -> V5/V6*in(ITC)/1, V5/V6*in(GL)/2
  out=ktsi*y(ITC)SI2/1 -> Out ITC/1, V5/V6*in-abs-out,ITC/2
  ktsi ITC/1 -> out=ktsi*y(ITC)SI2/1
  Integrator SI ITC2/1 -> out=ktsi*y(ITC)SI2/2, abs=ka*y(ITC)SI3/1, "ITC conc, y"/1  "ITC conc, y"
  Integrator SI GL2/1 -> "GL conc, y"/1, out=ktsi*y(GL)SI2/1  "GL conc, y"
  V5/V6*in-out,GL/1 -> Integrator SI GL2/1  "dy/dt SI GL"
  V5/V6*in(GL)/1 -> V5/V6*in-out,GL/1
  V5/V6*in(ITC)/1 -> V5/V6*in-abs-out,ITC/1
  V5/V6*in-abs-out,ITC/1 -> Integrator SI ITC2/1  "dy/dt SI  ITC"
  ka/1 -> abs=ka*y(ITC)SI3/2
  ktsi GL/1 -> out=ktsi*y(GL)SI2/2
  In ITC/1 -> V5/V6*in(ITC)/2
  In GL/1 -> V5/V6*in(GL)/1
  "V6=VSI/NSI, SI "/1 -> abs*V6/1
  SI Volume/1 -> "V6=VSI/NSI, SI "/1
  SI # compartments/1 -> "V6=VSI/NSI, SI "/2
  abs*V6/1 -> Gain/1
  Gain/1 -> abs/1

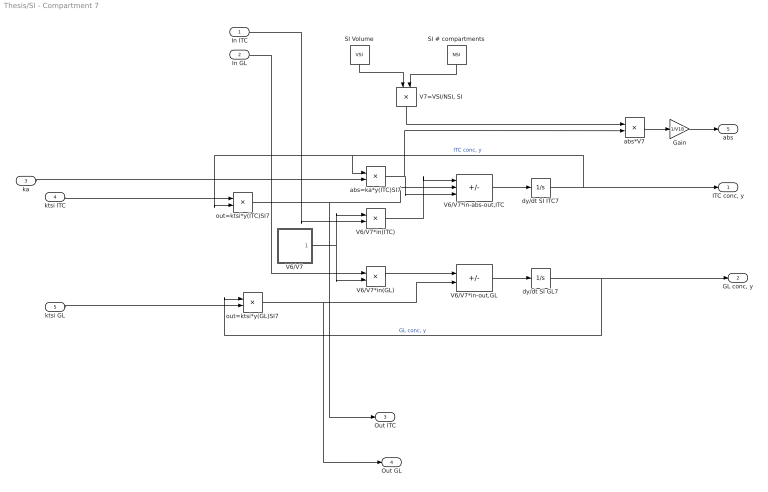
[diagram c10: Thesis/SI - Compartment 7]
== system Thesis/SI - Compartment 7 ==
  In ITC : Inport
  In GL : Inport  Port=2
  ka : Inport  Port=3
  ktsi ITC : Inport  Port=4
  ktsi GL : Inport  Port=5
  Gain : Gain  Gain=1/V18
  SI # compartments : Constant  Value=NSI
  SI Volume : Constant  Value=VSI
  V6/V7 : Subsystem
  V6/V7*in(GL) : Product
  V6/V7*in(ITC) : Product
  V6/V7*in-abs-out,ITC : Sum  Inputs=+--
  V6/V7*in-out,GL : Sum  Inputs=|+-
  "V7=VSI/NSI, SI " : Product  Inputs=*/
  abs*V7 : Product
  abs=ka*y(ITC)SI7 : Product
  dy/dt SI GL7 : Integrator
  dy/dt SI ITC7 : Integrator
  out=ktsi*y(GL)SI7 : Product
  out=ktsi*y(ITC)SI7 : Product
  "ITC conc, y" : Outport
  "GL conc, y" : Outport  Port=2
  Out ITC : Outport  Port=3
  Out GL : Outport  Port=4
  abs : Outport  Port=5
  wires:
  out=ktsi*y(GL)SI7/1 -> Out GL/1, V6/V7*in-out,GL/2
  V6/V7*in-abs-out,ITC/1 -> dy/dt SI ITC7/1
  dy/dt SI ITC7/1 -> abs=ka*y(ITC)SI7/1, out=ktsi*y(ITC)SI7/2, "ITC conc, y"/1  "ITC conc, y"
  V6/V7*in-out,GL/1 -> dy/dt SI GL7/1
  V6/V7/1(Out1) -> V6/V7*in(ITC)/1, V6/V7*in(GL)/2
  In ITC/1 -> V6/V7*in(ITC)/2
  out=ktsi*y(ITC)SI7/1 -> Out ITC/1, V6/V7*in-abs-out,ITC/2
  abs=ka*y(ITC)SI7/1 -> V6/V7*in-abs-out,ITC/3, abs*V7/2
  dy/dt SI GL7/1 -> out=ktsi*y(GL)SI7/1, "GL conc, y"/1  "GL conc, y"
  V6/V7*in(GL)/1 -> V6/V7*in-out,GL/1
  V6/V7*in(ITC)/1 -> V6/V7*in-abs-out,ITC/1
  In GL/1 -> V6/V7*in(GL)/1
  ka/1 -> abs=ka*y(ITC)SI7/2
  ktsi ITC/1 -> out=ktsi*y(ITC)SI7/1
  ktsi GL/1 -> out=ktsi*y(GL)SI7/2
  SI Volume/1 -> "V7=VSI/NSI, SI "/1
  SI # compartments/1 -> "V7=VSI/NSI, SI "/2
  "V7=VSI/NSI, SI "/1 -> abs*V7/1
  abs*V7/1 -> Gain/1
  Gain/1 -> abs/1

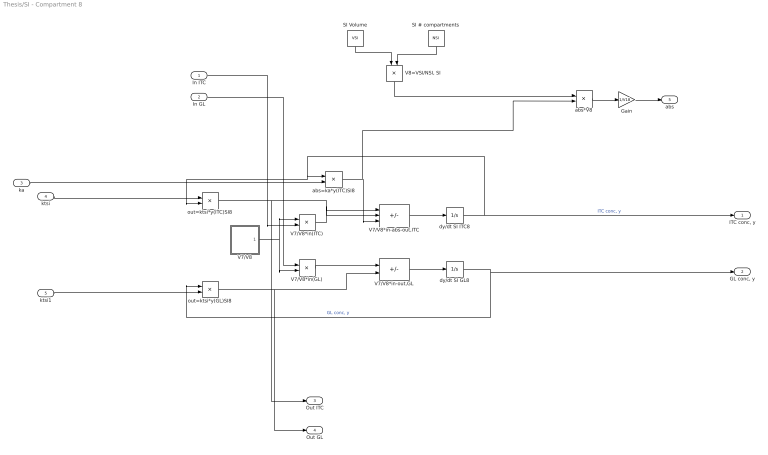
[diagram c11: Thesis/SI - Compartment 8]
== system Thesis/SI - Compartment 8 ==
  In ITC : Inport
  In GL : Inport  Port=2
  ka : Inport  Port=3
  ktsi : Inport  Port=4
  ktsi1 : Inport  Port=5
  Gain : Gain  Gain=1/V18
  SI # compartments : Constant  Value=NSI
  SI Volume : Constant  Value=VSI
  V7/V8 : Subsystem
  V7/V8*in(GL) : Product
  V7/V8*in(ITC) : Product
  V7/V8*in-abs-out,ITC : Sum  Inputs=+--
  V7/V8*in-out,GL : Sum  Inputs=|+-
  "V8=VSI/NSI, SI " : Product  Inputs=*/
  abs*V8 : Product
  abs=ka*y(ITC)SI8 : Product
  dy/dt SI GL8 : Integrator
  dy/dt SI ITC8 : Integrator
  out=ktsi*y(GL)SI8 : Product
  out=ktsi*y(ITC)SI8 : Product
  "ITC conc, y" : Outport
  "GL conc, y" : Outport  Port=2
  Out ITC : Outport  Port=3
  Out GL : Outport  Port=4
  abs : Outport  Port=5
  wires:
  V7/V8*in(GL)/1 -> V7/V8*in-out,GL/1
  dy/dt SI GL8/1 -> "GL conc, y"/1, out=ktsi*y(GL)SI8/1  "GL conc, y"
  In GL/1 -> V7/V8*in(GL)/1
  V7/V8*in(ITC)/1 -> V7/V8*in-abs-out,ITC/1
  dy/dt SI ITC8/1 -> out=ktsi*y(ITC)SI8/2, abs=ka*y(ITC)SI8/1, "ITC conc, y"/1  "ITC conc, y"
  V7/V8/1(Out1) -> V7/V8*in(GL)/2, V7/V8*in(ITC)/1
  abs=ka*y(ITC)SI8/1 -> abs*V8/2, V7/V8*in-abs-out,ITC/3
  ka/1 -> abs=ka*y(ITC)SI8/2
  out=ktsi*y(GL)SI8/1 -> Out GL/1, V7/V8*in-out,GL/2
  out=ktsi*y(ITC)SI8/1 -> Out ITC/1, V7/V8*in-abs-out,ITC/2
  V7/V8*in-abs-out,ITC/1 -> dy/dt SI ITC8/1
  V7/V8*in-out,GL/1 -> dy/dt SI GL8/1
  In ITC/1 -> V7/V8*in(ITC)/2
  ktsi/1 -> out=ktsi*y(ITC)SI8/1
  ktsi1/1 -> out=ktsi*y(GL)SI8/2
  SI Volume/1 -> "V8=VSI/NSI, SI "/1
  SI # compartments/1 -> "V8=VSI/NSI, SI "/2
  "V8=VSI/NSI, SI "/1 -> abs*V8/1
  abs*V8/1 -> Gain/1
  Gain/1 -> abs/1

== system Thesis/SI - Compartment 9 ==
  In ITC : Inport
  In GL : Inport  Port=2
  ka : Inport  Port=3
  ktsi : Inport  Port=4
  Gain : Gain  Gain=1/V18
  SI # compartments : Constant  Value=NSI
  SI Volume : Constant  Value=VSI
  V8/V9 : Subsystem
  V8/V9*in(GL) : Product
  V8/V9*in(ITC) : Product
  V8/V9*in-abs-out,ITC : Sum  Inputs=+--
  V8/V9*in-out,GL : Sum  Inputs=|+-
  "V9=VSI/NSI, SI " : Product  Inputs=*/
  abs*V9 : Product
  abs=ka*y(ITC)SI9 : Product
  dy/dt SI GL9 : Integrator
  dy/dt SI ITC9 : Integrator
  out=ktsi*y(GL)SI9 : Product
  out=ktsi*y(ITC)SI9 : Product
  "ITC conc, y" : Outport
  "GL conc, y" : Outport  Port=2
  Out ITC : Outport  Port=3
  Out GL : Outport  Port=4
  abs : Outport  Port=5
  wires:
  V8/V9*in-abs-out,ITC/1 -> dy/dt SI ITC9/1
  out=ktsi*y(ITC)SI9/1 -> Out ITC/1, V8/V9*in-abs-out,ITC/2
  out=ktsi*y(GL)SI9/1 -> Out GL/1, V8/V9*in-out,GL/2
  V8/V9/1(Out1) -> V8/V9*in(GL)/2, V8/V9*in(ITC)/1
  abs=ka*y(ITC)SI9/1 -> abs*V9/2, V8/V9*in-abs-out,ITC/3
  dy/dt SI ITC9/1 -> out=ktsi*y(ITC)SI9/2, abs=ka*y(ITC)SI9/1, "ITC conc, y"/1  "ITC conc, y"
  V8/V9*in(ITC)/1 -> V8/V9*in-abs-out,ITC/1
  In ITC/1 -> V8/V9*in(ITC)/2
  V8/V9*in(GL)/1 -> V8/V9*in-out,GL/1
  dy/dt SI GL9/1 -> "GL conc, y"/1, out=ktsi*y(GL)SI9/1  "GL conc, y"
  V8/V9*in-out,GL/1 -> dy/dt SI GL9/1
  ktsi/1 -> out=ktsi*y(GL)SI9/2, out=ktsi*y(ITC)SI9/1
  In GL/1 -> V8/V9*in(GL)/1
  ka/1 -> abs=ka*y(ITC)SI9/2
  SI Volume/1 -> "V9=VSI/NSI, SI "/1
  SI # compartments/1 -> "V9=VSI/NSI, SI "/2
  "V9=VSI/NSI, SI "/1 -> abs*V9/1
  abs*V9/1 -> Gain/1
  Gain/1 -> abs/1

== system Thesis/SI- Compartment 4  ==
  In ITC : Inport
  In GL : Inport  Port=2
  ktsi : Inport  Port=3
  Integrator Duodenum GL : Integrator
  Intregrator Duodenum ITC : Integrator
  V3/V4 : Subsystem
  V3/V4*in(GL) : Product
  V3/V4*in(ITC) : Product
  V3/V4*in-out,GL : Sum  Inputs=|+-
  V3/V4*in-out,ITC : Sum  Inputs=+-
  out=ktsi*y(GL) : Product
  out=ktsi*y(ITC) : Product
  "ITC conc, y" : Outport
  "GL conc, y" : Outport  Port=2
  Out ITC : Outport  Port=3
  Out GL : Outport  Port=4
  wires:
  Integrator Duodenum GL/1 -> "GL conc, y"/1, out=ktsi*y(GL)/1  "GL conc, y"
  ktsi/1 -> out=ktsi*y(GL)/2, out=ktsi*y(ITC)/1  "ktsi"
  V3/V4*in-out,GL/1 -> Integrator Duodenum GL/1  "dy/dt Duodenum GL"
  out=ktsi*y(ITC)/1 -> Out ITC/1, V3/V4*in-out,ITC/2
  Intregrator Duodenum ITC/1 -> "ITC conc, y"/1, out=ktsi*y(ITC)/2  "ITC conc, y"
  V3/V4/1(Out1) -> V3/V4*in(ITC)/1, V3/V4*in(GL)/2
  out=ktsi*y(GL)/1 -> Out GL/1, V3/V4*in-out,GL/2
  V3/V4*in-out,ITC/1 -> Intregrator Duodenum ITC/1  "dy/dt Duodenum ITC"
  V3/V4*in(ITC)/1 -> V3/V4*in-out,ITC/1
  V3/V4*in(GL)/1 -> V3/V4*in-out,GL/1
  In GL/1 -> V3/V4*in(GL)/1
  In ITC/1 -> V3/V4*in(ITC)/2

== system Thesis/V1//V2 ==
  Divide : Product  Inputs=*/
  V1 : Constant  Value=V1
  V2 : Constant  Value=V2
  Out1 : Outport
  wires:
  V1/1 -> Divide/1
  V2/1 -> Divide/2
  Divide/1 -> Out1/1

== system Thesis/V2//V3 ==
  Divide : Product  Inputs=*/
  V2 : Constant  Value=V2
  V3 : Constant  Value=V3
  Out1 : Outport
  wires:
  V2/1 -> Divide/1
  V3/1 -> Divide/2
  Divide/1 -> Out1/1

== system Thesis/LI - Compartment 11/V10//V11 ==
  Divide : Product  Inputs=*/
  LI # compartments : Constant  Value=NLI
  LI Volume : Constant  Value=VLI
  SI # compartments1 : Constant  Value=NSI
  SI Volume1 : Constant  Value=VSI
  V10=VSI/NSI : Product  Inputs=*/
  "V11=VLI/NLI " : Product  Inputs=*/
  Out1 : Outport
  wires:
  Divide/1 -> Out1/1
  LI Volume/1 -> "V11=VLI/NLI "/1
  LI # compartments/1 -> "V11=VLI/NLI "/2
  "V11=VLI/NLI "/1 -> Divide/2
  V10=VSI/NSI/1 -> Divide/1
  SI # compartments1/1 -> V10=VSI/NSI/2
  SI Volume1/1 -> V10=VSI/NSI/1

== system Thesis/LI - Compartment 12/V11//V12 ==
  Divide : Product  Inputs=*/
  LI # compartments : Constant  Value=NLI
  LI # compartments1 : Constant  Value=NLI
  LI Volume : Constant  Value=VLI
  LI Volume1 : Constant  Value=VLI
  V11=VLI/NLI : Product  Inputs=*/
  "V12=VLI/NLI " : Product  Inputs=*/
  Out1 : Outport
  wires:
  Divide/1 -> Out1/1
  LI Volume/1 -> "V12=VLI/NLI "/1
  LI # compartments/1 -> "V12=VLI/NLI "/2
  "V12=VLI/NLI "/1 -> Divide/2
  V11=VLI/NLI/1 -> Divide/1
  LI # compartments1/1 -> V11=VLI/NLI/2
  LI Volume1/1 -> V11=VLI/NLI/1

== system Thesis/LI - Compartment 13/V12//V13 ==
  Divide : Product  Inputs=*/
  LI # compartments : Constant  Value=NLI
  LI # compartments1 : Constant  Value=NLI
  LI Volume : Constant  Value=VLI
  LI Volume1 : Constant  Value=VLI
  V11=VLI/NLI : Product  Inputs=*/
  "V12=VLI/NLI " : Product  Inputs=*/
  Out1 : Outport
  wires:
  Divide/1 -> Out1/1
  LI Volume/1 -> "V12=VLI/NLI "/1
  LI # compartments/1 -> "V12=VLI/NLI "/2
  "V12=VLI/NLI "/1 -> Divide/2
  V11=VLI/NLI/1 -> Divide/1
  LI # compartments1/1 -> V11=VLI/NLI/2
  LI Volume1/1 -> V11=VLI/NLI/1

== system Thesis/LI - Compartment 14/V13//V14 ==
  Divide : Product  Inputs=*/
  LI # compartments : Constant  Value=NLI
  LI # compartments1 : Constant  Value=NLI
  LI Volume : Constant  Value=VLI
  LI Volume1 : Constant  Value=VLI
  V11=VLI/NLI : Product  Inputs=*/
  "V12=VLI/NLI " : Product  Inputs=*/
  Out1 : Outport
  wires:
  Divide/1 -> Out1/1
  LI Volume/1 -> "V12=VLI/NLI "/1
  LI # compartments/1 -> "V12=VLI/NLI "/2
  "V12=VLI/NLI "/1 -> Divide/2
  V11=VLI/NLI/1 -> Divide/1
  LI # compartments1/1 -> V11=VLI/NLI/2
  LI Volume1/1 -> V11=VLI/NLI/1

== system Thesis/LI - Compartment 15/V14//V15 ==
  Divide : Product  Inputs=*/
  LI # compartments : Constant  Value=NLI
  LI # compartments1 : Constant  Value=NLI
  LI Volume : Constant  Value=VLI
  LI Volume1 : Constant  Value=VLI
  V11=VLI/NLI : Product  Inputs=*/
  "V12=VLI/NLI " : Product  Inputs=*/
  Out1 : Outport
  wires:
  Divide/1 -> Out1/1
  LI Volume/1 -> "V12=VLI/NLI "/1
  LI # compartments/1 -> "V12=VLI/NLI "/2
  "V12=VLI/NLI "/1 -> Divide/2
  V11=VLI/NLI/1 -> Divide/1
  LI # compartments1/1 -> V11=VLI/NLI/2
  LI Volume1/1 -> V11=VLI/NLI/1

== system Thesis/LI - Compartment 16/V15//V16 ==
  Divide : Product  Inputs=*/
  LI # compartments : Constant  Value=NLI
  LI # compartments1 : Constant  Value=NLI
  LI Volume : Constant  Value=VLI
  LI Volume1 : Constant  Value=VLI
  V11=VLI/NLI : Product  Inputs=*/
  "V12=VLI/NLI " : Product  Inputs=*/
  Out1 : Outport
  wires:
  Divide/1 -> Out1/1
  LI Volume/1 -> "V12=VLI/NLI "/1
  LI # compartments/1 -> "V12=VLI/NLI "/2
  "V12=VLI/NLI "/1 -> Divide/2
  V11=VLI/NLI/1 -> Divide/1
  LI # compartments1/1 -> V11=VLI/NLI/2
  LI Volume1/1 -> V11=VLI/NLI/1

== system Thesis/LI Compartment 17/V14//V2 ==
  Divide : Product  Inputs=*/
  LI # compartments : Constant  Value=NLI
  LI # compartments1 : Constant  Value=NLI
  LI Volume : Constant  Value=VLI
  LI Volume1 : Constant  Value=VLI
  V11=VLI/NLI : Product  Inputs=*/
  "V12=VLI/NLI " : Product  Inputs=*/
  Out1 : Outport
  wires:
  Divide/1 -> Out1/1
  LI Volume/1 -> "V12=VLI/NLI "/1
  LI # compartments/1 -> "V12=VLI/NLI "/2
  "V12=VLI/NLI "/1 -> Divide/2
  V11=VLI/NLI/1 -> Divide/1
  LI # compartments1/1 -> V11=VLI/NLI/2
  LI Volume1/1 -> V11=VLI/NLI/1

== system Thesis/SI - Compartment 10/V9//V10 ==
  Divide : Product  Inputs=*/
  SI # compartments : Constant  Value=NSI
  SI # compartments1 : Constant  Value=NSI
  SI Volume : Constant  Value=VSI
  SI Volume1 : Constant  Value=VSI
  "V8=VSI/NSI, SI 1" : Product  Inputs=*/
  "V9=VSI/NSI, SI " : Product  Inputs=*/
  Out1 : Outport
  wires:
  Divide/1 -> Out1/1
  SI Volume/1 -> "V9=VSI/NSI, SI "/1
  SI # compartments/1 -> "V9=VSI/NSI, SI "/2
  "V9=VSI/NSI, SI "/1 -> Divide/2  "V9"
  "V8=VSI/NSI, SI 1"/1 -> Divide/1  "V8"
  SI # compartments1/1 -> "V8=VSI/NSI, SI 1"/2
  SI Volume1/1 -> "V8=VSI/NSI, SI 1"/1

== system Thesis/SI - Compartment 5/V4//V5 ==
  Divide : Product  Inputs=*/
  SI # compartments : Constant  Value=NSI
  SI Volume : Constant  Value=VSI
  V4 : Constant  Value=V4
  "V5=VSI/NSI, SI " : Product  Inputs=*/
  Out1 : Outport
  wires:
  V4/1 -> Divide/1
  Divide/1 -> Out1/1
  SI Volume/1 -> "V5=VSI/NSI, SI "/1
  SI # compartments/1 -> "V5=VSI/NSI, SI "/2
  "V5=VSI/NSI, SI "/1 -> Divide/2

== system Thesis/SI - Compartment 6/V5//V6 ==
  Divide : Product  Inputs=*/
  SI # compartments : Constant  Value=NSI
  SI # compartments1 : Constant  Value=NSI
  SI Volume : Constant  Value=VSI
  SI Volume1 : Constant  Value=VSI
  "V5=VSI/NSI, SI 1" : Product  Inputs=*/
  "V6=VSI/NSI, SI " : Product  Inputs=*/
  Out1 : Outport
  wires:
  Divide/1 -> Out1/1
  SI Volume/1 -> "V6=VSI/NSI, SI "/1
  SI # compartments/1 -> "V6=VSI/NSI, SI "/2
  "V6=VSI/NSI, SI "/1 -> Divide/2  "V6"
  "V5=VSI/NSI, SI 1"/1 -> Divide/1  "V5"
  SI # compartments1/1 -> "V5=VSI/NSI, SI 1"/2
  SI Volume1/1 -> "V5=VSI/NSI, SI 1"/1

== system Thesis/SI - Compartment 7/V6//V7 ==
  Divide : Product  Inputs=*/
  SI # compartments : Constant  Value=NSI
  SI # compartments1 : Constant  Value=NSI
  SI Volume : Constant  Value=VSI
  SI Volume1 : Constant  Value=VSI
  "V6=VSI/NSI, SI 1" : Product  Inputs=*/
  "V7=VSI/NSI, SI " : Product  Inputs=*/
  Out1 : Outport
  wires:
  Divide/1 -> Out1/1
  SI Volume/1 -> "V7=VSI/NSI, SI "/1
  SI # compartments/1 -> "V7=VSI/NSI, SI "/2
  "V7=VSI/NSI, SI "/1 -> Divide/2  "V7"
  "V6=VSI/NSI, SI 1"/1 -> Divide/1  "V6"
  SI # compartments1/1 -> "V6=VSI/NSI, SI 1"/2
  SI Volume1/1 -> "V6=VSI/NSI, SI 1"/1

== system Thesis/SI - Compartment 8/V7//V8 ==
  Divide : Product  Inputs=*/
  SI # compartments : Constant  Value=NSI
  SI # compartments1 : Constant  Value=NSI
  SI Volume : Constant  Value=VSI
  SI Volume1 : Constant  Value=VSI
  "V7=VSI/NSI, SI 1" : Product  Inputs=*/
  "V8=VSI/NSI, SI " : Product  Inputs=*/
  Out1 : Outport
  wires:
  Divide/1 -> Out1/1
  SI Volume/1 -> "V8=VSI/NSI, SI "/1
  SI # compartments/1 -> "V8=VSI/NSI, SI "/2
  "V8=VSI/NSI, SI "/1 -> Divide/2  "V8"
  "V7=VSI/NSI, SI 1"/1 -> Divide/1  "V7"
  SI # compartments1/1 -> "V7=VSI/NSI, SI 1"/2
  SI Volume1/1 -> "V7=VSI/NSI, SI 1"/1
